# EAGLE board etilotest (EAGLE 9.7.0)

Size 208.49 x 164.85 mm. Coordinates in mm from the lower left corner, seen from the top.
Outline: 0,0 208.49,0 208.49,164.84 0,164.84 0,0
Copper layers (1*16): Top 0.035mm / dielectric 1.5mm / Bottom 0.035mm
Design rules "default": minimum track width 6mil, minimum drill 0.35mm, track to track 6mil, track to pad 6mil, pad to pad 6mil, via to via 6mil, smd to smd 6mil, copper to edge 40mil, drill to drill 6mil, minimum pad ring 10mil, minimum via ring 8mil, stop-mask expansion 4mil, vias tented up to drill 0mil, thermal gap 10mil

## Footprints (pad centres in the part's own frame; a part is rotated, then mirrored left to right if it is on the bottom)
MQ-XX-SOCKET = drill 1.27: 1 -6.223,6.223; 2 -8.788,0; 3 -6.223,-6.223; 4 6.223,-6.223; 5 8.788,0; 6 6.223,6.223
PIEZO = drill 1 pad 1.6: 1 -3.5,0; 2 3.5,0
RESAD1016W63L850D250B = drill 0.83 pad 1.43: 1 -5.08,0; 2 5.08,0
SWITCH-MOMENTARY-PTH-6.5MM = drill 1.016 pad 1.88: 1 -3.251,2.261; 2 3.251,2.261; 3 -3.251,-2.261; 4 3.251,-2.261
ARDUINO-UNO-R3-SHIELD = drill 1.016 pad 1.88: 3.3V 24.13,-2.54; 5V 24.13,0; A0 24.13,12.7; A1 24.13,15.24; A2 24.13,17.78; A3 24.13,20.32; A4 24.13,22.86; A5 24.13,25.4; AREF -24.13,-13.97; D2 -24.13,20.32; D3 -24.13,17.78; D4 -24.13,15.24; D5 -24.13,12.7; D6 -24.13,10.16; D7 -24.13,7.62; D8 -24.13,3.81; D9 -24.13,1.27; D10 -24.13,-1.27; D11 -24.13,-3.81; D12 -24.13,-6.35; D13 -24.13,-8.89; GND@0 24.13,2.54; GND@1 24.13,5.08; GND@2 -24.13,-11.43; IOREF 24.13,-7.62; NC 24.13,-10.16; RES 24.13,-5.08; RX -24.13,25.4; SCL -24.13,-19.05; SDA -24.13,-16.51; TX -24.13,22.86; VIN 24.13,7.62
LCD-I2C = drill 1.016 long: 1 -19.05,-5.08; 2 -19.05,-7.62; 3 -19.05,-10.16; 4 -19.05,-12.7

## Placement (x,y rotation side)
GAS1  GAS-SENSORMQ-XX-SOCKET  [MQ-XX-SOCKET]  14.22,123.5 270 top
PIEZO1  PIEZO  [PIEZO]  168.38,114.81 270 top
R1  1k  [RESAD1016W63L850D250B]  46.37,109.07 0 top
S1  SWITCH_MOMENTARY  [SWITCH-MOMENTARY-PTH-6.5MM]  200.24,82.86 90 top
U1  ARDUINO-UNO-R3-SHIELD  [ARDUINO-UNO-R3-SHIELD]  119.2,116.96 180 top
U2  LCD-16X2-I2CSUNFOUNDER-IIC  [LCD-I2C]  106.69,36.63 0 top

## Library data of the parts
GAS1 PIEZO1 R1 S1 U1 U2 = Tinkercad

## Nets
U1_5V: GAS1.1 GAS1.3 U1.5V U2.2
U1_A4: U1.A4 U2.3
U1_A5: U1.A5 U2.4
U1_D4: S1.2 U1.D4
U1_D11: PIEZO1.1 U1.D11
U1_GND: GAS1.5 PIEZO1.2 R1.1 R1.2 S1.3 U1.A1 U1.GND@0 U1.GND@1 U1.GND@2 U2.1
U1_VIN: GAS1.2 U1.VIN

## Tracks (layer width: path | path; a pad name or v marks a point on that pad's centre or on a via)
U1_5V  (3 unrouted)
U1_A4  (1 unrouted)
U1_A5  (1 unrouted)
U1_D4  (1 unrouted)
U1_D11  (1 unrouted)
U1_GND  (9 unrouted)
U1_VIN  (1 unrouted)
